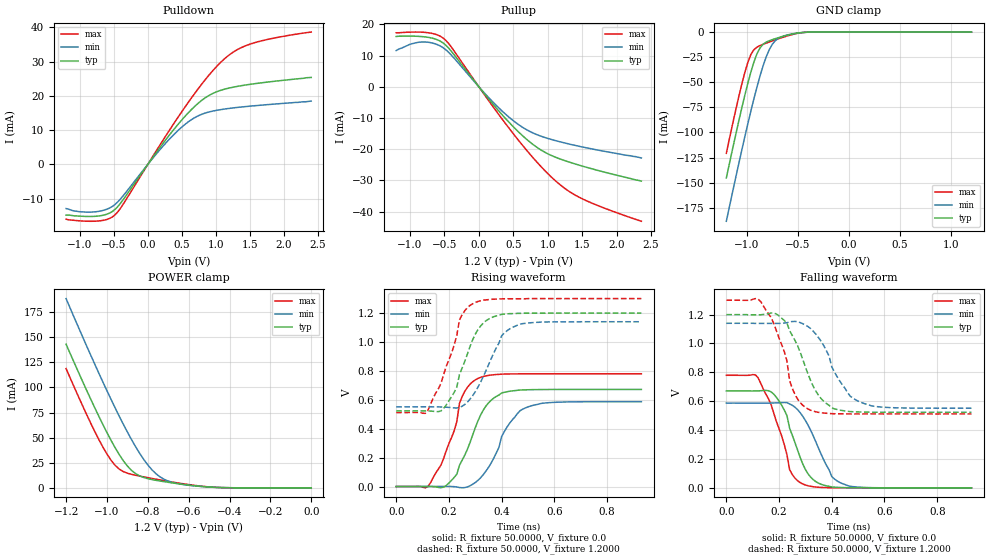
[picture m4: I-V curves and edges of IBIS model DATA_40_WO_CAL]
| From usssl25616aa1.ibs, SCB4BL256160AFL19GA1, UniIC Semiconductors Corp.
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|   Model DATA_40_WO_CAL
[Model]  DATA_40_WO_CAL
Model_type I/O
Polarity   Non-Inverting
Enable   Active-High
Vinl =   0.3800V
Vinh =   0.8200V
Vmeas =  0.6000V
Cref =   5.0000pF
Rref =   50.0000
Vref =   0.6000V
C_comp   1.7430pF   1.7110pF   1.7640pF
[Temperature Range]   25.0000   0.1250k   -40.0000
[Voltage Range]   1.2000V   1.1400V   1.3000V
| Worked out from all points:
|   slope of the pulldown table from 0 to 0.18 V, typ, clamps not added: 36.2 ohm
|   slope of the pullup table from 0 to 0.18 V, typ, clamps not added: 36.7 ohm
|   GND clamp passes 1 mA (typ) near -0.50 V on its own axis
|   POWER clamp passes 1 mA (typ) near -0.51 V on its own axis
|   rising waveform, R_fixture 50.0000, V_fixture 0.0: 20-80 % time 95.4ps typ, 100ps min, 79.3ps max; typ from 0 V to 0.672 V
|   rising waveform, R_fixture 50.0000, V_fixture 1.2000: 20-80 % time 81.5ps typ, 91.5ps min, 81.3ps max; typ from 0.523 V to 1.2 V
|   falling waveform, R_fixture 50.0000, V_fixture 0.0: 20-80 % time 77.9ps typ, 92.6ps min, 79.3ps max; typ from 0.672 V to 0 V
|   falling waveform, R_fixture 50.0000, V_fixture 1.2000: 20-80 % time 96.1ps typ, 100ps min, 75.8ps max; typ from 1.2 V to 0.523 V
[Pulldown]
|Voltage   I(typ)   I(min)   I(max)
-1.2V     -14.8mA    -12.9mA    -16mA
-800mV    -15.19mA   -13.89mA   -16.6mA
-600mV    -14.54mA   -13.08mA   -16.08mA
-480mV    -13.11mA   -11.68mA   -14.71mA
-360mV    -10.25mA   -9.116mA   -11.57mA
200mV     5.517mA    4.805mA    6.349mA
520mV     13.45mA    11.26mA    16mA
840mV     19.41mA    14.98mA    24.66mA
1.2V      22.33mA    16.37mA    32.04mA
1.36V     22.95mA    16.74mA    33.99mA
1.6V      23.66mA    17.19mA    35.73mA
2.4V      25.4mA     18.5mA     38.66mA
[Pullup]
|Voltage   I(typ)   I(min)   I(max)
-1.2V     16.1mA     11.6mA     17.3mA
-840mV    16.09mA    14.33mA    17.5mA
-680mV    15.59mA    14.04mA    17.1mA
-520mV    14.05mA    12.53mA    15.63mA
-400mV    11.39mA    10.15mA    12.74mA
80mV      -2.217mA   -1.976mA   -2.506mA
360mV     -9.503mA   -8.228mA   -10.99mA
600mV     -14.97mA   -12.48mA   -17.81mA
840mV     -19.35mA   -15.31mA   -24.06mA
1.12V     -22.63mA   -17.29mA   -30.27mA
1.4V      -24.74mA   -18.8mA    -34.72mA
2.36V     -30.2mA    -22.8mA    -43.09mA
[GND_clamp]
|Voltage   I(typ)   I(min)   I(max)
-1.2V     -145.3mA   -188.5mA   -120.8mA
-1.05V    -76.2mA    -118.2mA   -52.43mA
-990mV    -51.2mA    -91.62mA   -30.39mA
-960mV    -39.9mA    -78.82mA   -22.48mA
-900mV    -21.67mA   -54.7mA    -15mA
-870mV    -15.78mA   -43.66mA   -13.45mA
-810mV    -10.04mA   -24.79mA   -11.07mA
-780mV    -8.658mA   -17.59mA   -9.958mA
-720mV    -6.57mA    -8.545mA   -7.793mA
-630mV    -3.906mA   -3.64mA    -4.741mA
-420mV    -215.4uA   -240.5uA   -235uA
1.2V      1.597nA    22.84nA    1.463nA
[POWER_clamp]
|Voltage   I(typ)   I(min)   I(max)
-1.2V     143mA      188.4mA    118.7mA
-1.1V     97.38mA    141.5mA    73.24mA
-1.04V    71.38mA    114.3mA    48.22mA
-1V       55.04mA    96.69mA    33.64mA
-960mV    40mA       79.65mA    22.42mA
-900mV    21.75mA    55.6mA     14.58mA
-860mV    14.17mA    41.05mA    12.52mA
-800mV    9.133mA    22.79mA    10.12mA
-740mV    6.786mA    10.88mA    7.886mA
-660mV    4.332mA    4.436mA    5.101mA
-520mV    1.103mA    1.063mA    1.274mA
0V        1.597nA    6.003nA    2.16nA
[Ramp]
| variable   typ   min   max
dV/dt_r  0.4030/90.3786p   0.3523/0.1024n   0.4679/83.0159p
dV/dt_f  0.4060/89.3830p   0.3531/0.1052n   0.4729/79.8092p
R_load = 50.0000
[Rising Waveform]
R_fixture= 50.0000
V_fixture= 0.0
V_fixture_min= 0.0
V_fixture_max= 0.0
|time   V(typ)   V(min)   V(max)
0s        0V         0V         0V
120ps     1.042mV    147uV      -141.5uV
170ps     -7.981mV   928uV      149.9mV
230ps     85.52mV    -2.621mV   450.3mV
250ps     182mV      -8.259mV   621.6mV
310ps     453.7mV    42.56mV    747.5mV
370ps     611.7mV    196.2mV    773.3mV
410ps     651.9mV    380.1mV    778.1mV
480ps     668.3mV    535.1mV    779.6mV
930ps     671.6mV    587.2mV    779.8mV
[Rising Waveform]
R_fixture= 50.0000
V_fixture= 1.2000
V_fixture_min= 1.1400
V_fixture_max= 1.3000
|time   V(typ)   V(min)   V(max)
0s        523.4mV    551.5mV    511.9mV
110ps     523.3mV    551.8mV    506.1mV
180ps     539.9mV    549.6mV    774.1mV
230ps     688.5mV    543.1mV    1.047V
240ps     775.7mV    547.6mV    1.153V
300ps     1.054V     655.8mV    1.273V
340ps     1.146V     799.8mV    1.291V
400ps     1.191V     1.043V     1.298V
460ps     1.198V     1.117V     1.299V
930ps     1.2V       1.14V      1.3V
[Falling Waveform]
R_fixture= 50.0000
V_fixture= 0.0
V_fixture_min= 0.0
V_fixture_max= 0.0
|time   V(typ)   V(min)   V(max)
0s        671.6mV    587.2mV    779.8mV
120ps     671.8mV    586.9mV    763.9mV
170ps     664.7mV    587.5mV    574.8mV
210ps     571.5mV    590.7mV    359.3mV
240ps     413.2mV    581.2mV    126.3mV
290ps     165mV      495.6mV    26.55mV
330ps     56.08mV    358.8mV    7.523mV
400ps     5.96mV     77.94mV    598.4uV
440ps     1.927mV    29.35mV    168uV
930ps     0V         0V         0V
[Falling Waveform]
R_fixture= 50.0000
V_fixture= 1.2000
V_fixture_min= 1.1400
V_fixture_max= 1.3000
|time   V(typ)   V(min)   V(max)
0s        1.2V       1.14V      1.3V
130ps     1.199V     1.139V     1.291V
180ps     1.211V     1.139V     1.139V
230ps     1.141V     1.144V     877.9mV
240ps     1.089V     1.15V      743.4mV
260ps     1.023V     1.153V     648.5mV
310ps     787.6mV    1.117V     546.1mV
400ps     553.8mV    838mV      513.9mV
500ps     525.8mV    600.7mV    512mV
930ps     523.4mV    551.5mV    511.9mV
